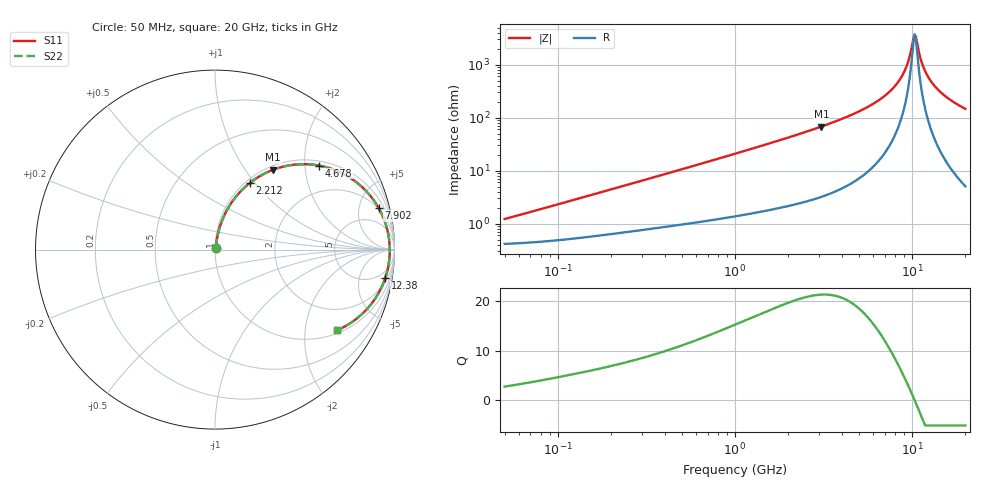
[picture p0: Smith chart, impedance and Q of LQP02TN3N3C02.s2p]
!Murata Part Number: LQP02TN3N3C02
!These Parameters are Measured in Series Mode Connection
!  o--[Z]--o
!Port1  Port2
!  o-------o
!Freq. Start=50[MHz] Stop=20[GHz], 401[Steps]
# Hz S RI R 50
!Freq.(Hz) S11(Real) S11(Imag) S21(Real) S21(Imag) S12(Real) S12(Imag) S22(Real) S22(Imag)
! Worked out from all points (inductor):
!   401 points, 50 MHz to 20 GHz, reference 50 ohm
!   read as one part in series: L = 3.65 nH near 55.53 MHz
!   highest Q = 21.2 at 3.075 GHz (marker M1), where L = 3.52 nH
!   self-resonance near 10.35 GHz
!   S11 on the Smith chart (normalised r, x): 50 MHz: 1.01, +0.02; 2.212 GHz: 1.05, +0.94; 4.678 GHz: 1.12, +2.36; 7.902 GHz: 1.86, +7.49; 12.38 GHz: 3, -11; 20 GHz: 1.10, -2.94
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5e7  0.00427 0.0114  0.9957 -0.0114  0.9957 -0.0114  0.00427 0.0114
1.364002e8  0.00634 0.0302  0.9937 -0.0302  0.9937 -0.0302  0.00634 0.0302
3.721004e8  0.0145 0.0778  0.9855 -0.0778  0.9855 -0.0778  0.0145 0.0778
1e9  0.0536 0.1946  0.9464 -0.1946  0.9464 -0.1946  0.0536 0.1946
2.211938e9  0.1929 0.3705  0.8071 -0.3705  0.8071 -0.3705  0.1929 0.3705
2.728004e9  0.2696 0.4205  0.7304 -0.4205  0.7304 -0.4205  0.2696 0.4205
3.075291e9  0.3244 0.4451  0.6756 -0.4451  0.6756 -0.4451  0.3244 0.4451
4.677679e9  0.5783 0.4686  0.4217 -0.4686  0.4217 -0.4686  0.5783 0.4686
6.125241e9  0.7663 0.3912  0.2337 -0.3912  0.2337 -0.3912  0.7663 0.3912
7.442007e9  0.8827 0.2773  0.1173 -0.2773  0.1173 -0.2773  0.8827 0.2773
7.901521e9  0.9111 0.2332  0.0889 -0.2332  0.0889 -0.2332  0.9111 0.2332
8.644534e9  0.9446 0.1607  0.0554 -0.1607  0.0554 -0.1607  0.9446 0.1607
9.178299e9  0.9603 0.109  0.0397 -0.109  0.0397 -0.109  0.9603 0.109
9.600142e9  0.9682 0.0691  0.0318 -0.0691  0.0318 -0.0691  0.9682 0.0691
1.004137e10  0.9727 0.0284  0.0273 -0.0284  0.0273 -0.0284  0.9727 0.0284
1.034674e10  0.9738 0.0011  0.0262 -0.0011  0.0262 -0.0011  0.9738 0.0011
1.066139e10  0.9734 -0.0262  0.0266 0.0262  0.0266 0.0262  0.9734 -0.0262
1.149051e10  0.9655 -0.0941  0.0345 0.0941  0.0345 0.0941  0.9655 -0.0941
1.238412e10  0.9482 -0.1598  0.0518 0.1598  0.0518 0.1598  0.9482 -0.1598
1.354865e10  0.916 -0.2338  0.084 0.2338  0.084 0.2338  0.916 -0.2338
1.504638e10  0.8647 -0.3105  0.1353 0.3105  0.1353 0.3105  0.8647 -0.3105
2e10  0.6777 -0.4504  0.3223 0.4504  0.3223 0.4504  0.6777 -0.4504
